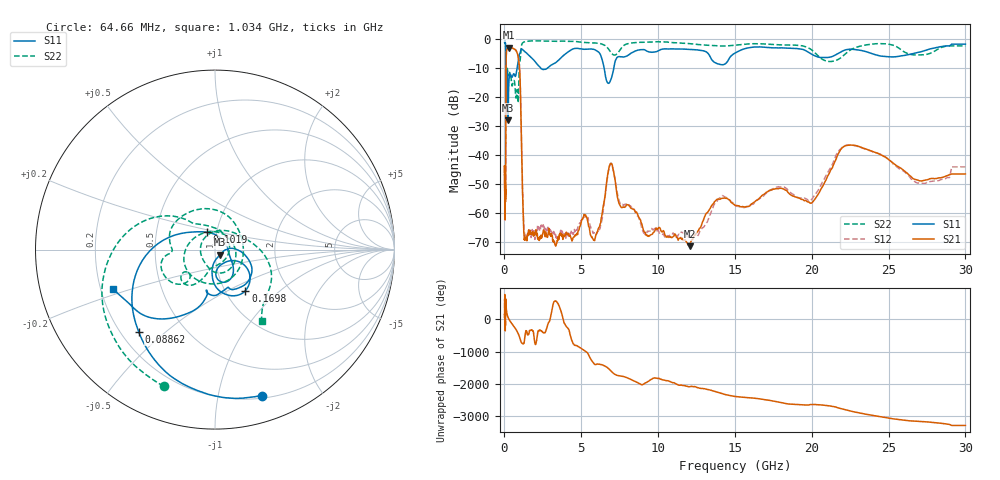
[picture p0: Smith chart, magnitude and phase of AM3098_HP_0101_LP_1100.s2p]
! Date/Time: Thu, Feb 28, 2019 8:36 AM
! Network Analyzer: Agilent Technologies E8364B Rev: A.07.50.67
! Sweep from 0.010 to 30.000 GHz, 1601 Points, Sweep Type: LOG
! Power Supply: 5.022 V, 0.002 A
# Hz S DB R 50
!freq MagS11 AngS11 MagS21 AngS21 MagS12 AngS12 MagS22 AngS22
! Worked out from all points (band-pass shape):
!   1601 points, 10 MHz to 30 GHz, reference 50 ohm
!   highest |S21| = -2.81 dB at 291.6 MHz (marker M1); lowest = -71.3 dB at 12.07 GHz (marker M2)
!   |S21| within 3 dB of the highest: 114.3 MHz to 888.3 MHz (774.1 MHz wide, 154 % of centre)
!   lowest |S11| = -27.9 dB at 236.3 MHz (marker M3), VSWR 1.08, Z = 52.9 - j2.93 ohm
!   |S11| at or under -10 dB: 97.45 MHz to 811.4 MHz (714 MHz wide, 157 % of centre); 2.376 GHz to 2.771 GHz (394.6 MHz wide, 15.3 % of centre); 6.494 GHz to 7.112 GHz (618.1 MHz wide, 9.09 % of centre)
!   |S22| runs from -22.2 to -0.5 dB; largest |S21 - S12| = 0.013
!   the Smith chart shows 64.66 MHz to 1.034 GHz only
!   S11 on the Smith chart (normalised r, x): 64.66 MHz: 0.22, -1.35; 88.62 MHz: 0.27, -0.41; 101.9 MHz: 0.90, +0.18; 169.8 MHz: 1.24, -0.62; 1.034 GHz: 0.25, -0.18
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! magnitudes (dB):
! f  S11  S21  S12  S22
! 10 MHz  -0.3  -43.6  -43.7  -0.6
! 38.04 MHz  -0.5  -59.6  -59.6  -1.0
! 64.66 MHz  -1.4  -54.8  -52.4  -1.8
! 88.62 MHz  -4.1  -36.1  -36.0  -4.5
! 101.9 MHz  -19.4  -11.4  -11.4  -21.6
! 144.7 MHz  -17.6  -3.7  -3.6  -13.7
! 169.8 MHz  -10.9  -3.4  -3.4  -10.2
! 236.3 MHz  -27.9  -2.9  -2.9  -12.2
! 291.6 MHz  -14.4  -2.8  -2.8  -12.0
! 550.5 MHz  -12.3  -3.1  -3.0  -14.9
! 885.5 MHz  -7.8  -5.7  -5.7  -21.7
! 1.034 GHz  -4.3  -16.7  -16.7  -6.5
! 1.282 GHz  -4.0  -68.3  -65.6  -0.9
! 2.084 GHz  -8.2  -66.3  -65.5  -0.5
! 5.841 GHz  -3.5  -69.3  -66.7  -1.2
! 6.924 GHz  -13.9  -42.8  -42.6  -4.5
! 7.926 GHz  -5.8  -57.2  -56.8  -1.6
! 12.07 GHz  -3.4  -71.3  -67.6  -1.4
! 14.02 GHz  -8.6  -55.1  -54.6  -2.2
! 19.9 GHz  -4.8  -56.4  -55.6  -3.3
! 22.56 GHz  -3.4  -36.4  -36.4  -3.5
! 30 GHz  -1.6  -46.4  -43.9  -2.2
